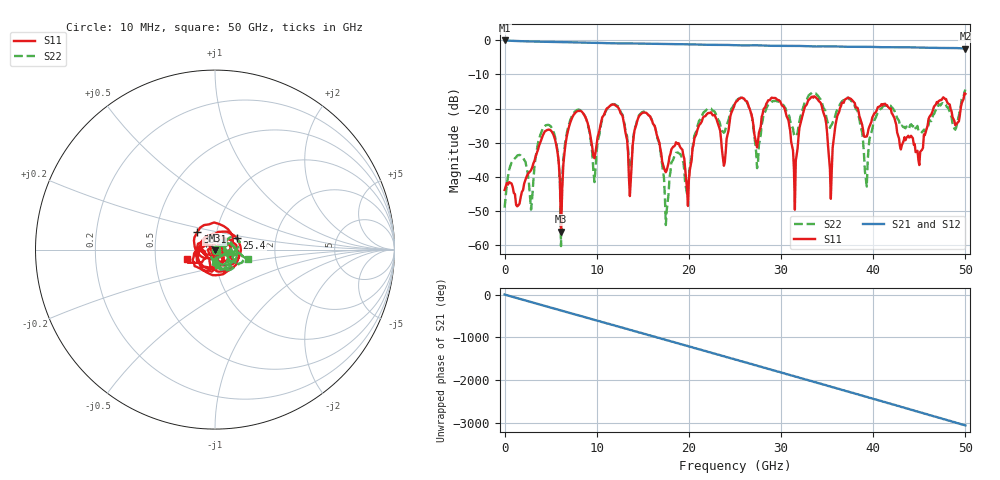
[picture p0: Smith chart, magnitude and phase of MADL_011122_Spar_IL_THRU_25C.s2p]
#	HZ	S	DB	R	50
!Frequency	S11 (dB)	S11-Ang	S21 (dB)	S21-Ang	S12 (dB)	S12-Ang	S22 (dB)	S22-Ang
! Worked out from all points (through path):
!   401 points, 10 MHz to 50 GHz, reference 50 ohm
!   highest |S21| = -0.01 dB at 10 MHz (marker M1); lowest = -2.4 dB at 50 GHz (marker M2)
!   group delay of S21, straight-line fit = 169 ps
!   lowest |S11| = -56.1 dB at 6.13 GHz (marker M3), VSWR 1.00, Z = 50 - j0.156 ohm
!   |S11| at or under -10 dB: start of sweep to end of sweep
!   |S22| runs from -60.4 to -14.4 dB; largest |S21 - S12| = 0.017
!   S11 on the Smith chart (normalised r, x): 10 MHz: 1.01, -0.01; 25.4 GHz: 1.27, +0.17; 33.1 GHz: 0.81, +0.16; 50 GHz: 0.73, -0.08
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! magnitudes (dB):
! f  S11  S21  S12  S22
! 10 MHz  -43.9  0.0  0.0  -49.1
! 4.63 GHz  -26.3  -0.4  -0.4  -24.8
! 6.13 GHz  -56.1  -0.5  -0.5  -60.4
! 8.38 GHz  -20.9  -0.7  -0.7  -20.8
! 9.76 GHz  -34.6  -0.7  -0.7  -41.6
! 11.6 GHz  -18.9  -0.8  -0.9  -18.9
! 13.6 GHz  -45.7  -0.9  -0.9  -37.6
! 16.8 GHz  -30.0  -1.0  -1.0  -30.2
! 17.6 GHz  -38.1  -1.1  -1.1  -49.8
! 25.1 GHz  -18.1  -1.4  -1.4  -17.8
! 25.4 GHz  -17.2  -1.4  -1.5  -17.1
! 27.4 GHz  -31.4  -1.4  -1.4  -37.5
! 29.8 GHz  -17.6  -1.6  -1.6  -18.0
! 31.5 GHz  -49.7  -1.6  -1.6  -28.2
! 33.1 GHz  -17.2  -1.8  -1.8  -15.9
! 33.4 GHz  -16.5  -1.8  -1.8  -15.3
! 35.4 GHz  -46.5  -1.8  -1.8  -25.0
! 37 GHz  -17.2  -1.9  -1.9  -17.2
! 39.3 GHz  -28.2  -1.9  -1.9  -42.9
! 41.8 GHz  -20.0  -2.0  -2.0  -19.2
! 44.9 GHz  -35.0  -2.1  -2.1  -26.5
! 50 GHz  -15.7  -2.4  -2.4  -14.4
